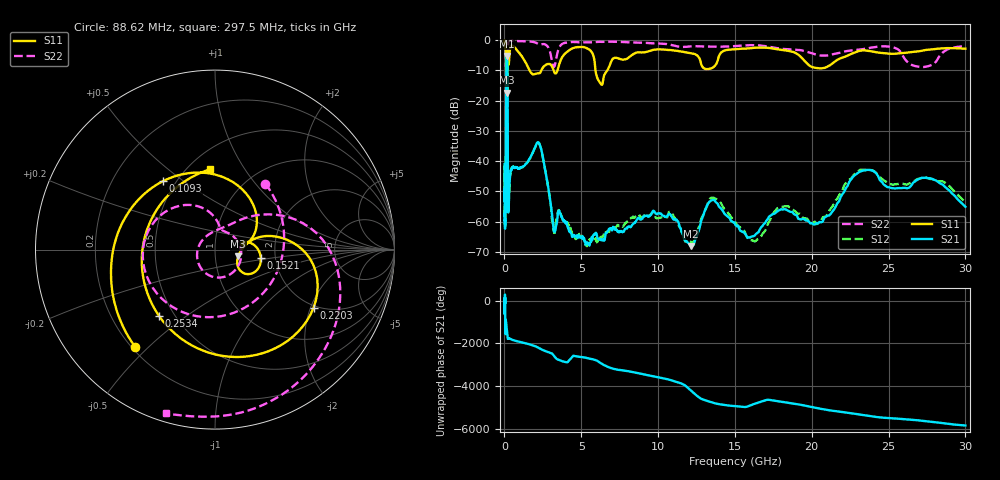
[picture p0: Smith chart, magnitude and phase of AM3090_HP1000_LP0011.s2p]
! Date/Time: Thu, Feb 28, 2019 2:01 PM
! Network Analyzer: Agilent Technologies E8364B Rev: A.07.50.67
! Sweep from 0.010 to 30.000 GHz, 1601 Points, Sweep Type: LOG
! Power Supply: 5.023 V, 0.002 A
# Hz S DB R 50
!freq MagS11 AngS11 MagS21 AngS21 MagS12 AngS12 MagS22 AngS22
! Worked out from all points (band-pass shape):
!   1601 points, 10 MHz to 30 GHz, reference 50 ohm
!   highest |S21| = -5.32 dB at 149.9 MHz (marker M1); lowest = -68.0 dB at 12.13 GHz (marker M2)
!   |S21| within 3 dB of the highest: 121.5 MHz to 190.9 MHz (69.33 MHz wide, 44.4 % of centre)
!   lowest |S11| = -17.4 dB at 185.8 MHz (marker M3), VSWR 1.31, Z = 64.7 - j4.81 ohm
!   |S11| at or under -10 dB: 1.623 GHz to 2.401 GHz (778.5 MHz wide, 38.7 % of centre); 3.196 GHz to 3.454 GHz (258 MHz wide, 7.76 % of centre); 5.925 GHz to 6.698 GHz (772.4 MHz wide, 12.2 % of centre)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
!   |S22| runs from -21.1 to -0.2 dB; largest |S21 - S12| = 0.013
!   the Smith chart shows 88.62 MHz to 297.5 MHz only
!   S11 on the Smith chart (normalised r, x): 88.62 MHz: 0.21, -0.45; 109.3 MHz: 0.43, +0.42; 152.1 MHz: 1.68, -0.17; 220.3 MHz: 1.93, -2.10; 253.4 MHz: 0.41, -0.40; 297.5 MHz: 0.63, +0.71
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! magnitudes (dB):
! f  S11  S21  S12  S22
! 10 MHz  -0.3  -41.0  -43.1  -0.6
! 38.04 MHz  -0.5  -60.2  -58.7  -1.4
! 88.62 MHz  -3.1  -48.6  -49.8  -6.7
! 109.3 MHz  -6.4  -19.1  -19.1  -7.8
! 144.7 MHz  -12.8  -5.4  -5.3  -17.3
! 149.9 MHz  -11.9  -5.3  -5.3  -16.4
! 152.1 MHz  -11.7  -5.3  -5.3  -16.1
! 185.8 MHz  -17.4  -7.2  -7.2  -20.3
! 201.3 MHz  -10.8  -14.3  -14.3  -11.5
! 220.3 MHz  -3.9  -43.6  -43.3  -2.8
! 253.4 MHz  -6.3  -56.0  -54.5  -0.8
! 297.5 MHz  -7.0  -51.5  -51.9  -0.4
! 550.5 MHz  -2.0  -41.9  -42.1  -0.3
! 2.084 GHz  -11.1  -34.3  -34.4  -1.0
! 3.204 GHz  -10.1  -62.9  -62.6  -8.9
! 7.926 GHz  -6.3  -62.3  -60.3  -0.7
! 12.13 GHz  -4.4  -68.0  -66.6  -2.1
! 13.61 GHz  -8.9  -52.9  -52.1  -2.2
! 16.21 GHz  -2.6  -64.8  -66.3  -1.7
! 20.41 GHz  -9.3  -60.6  -60.5  -5.0
! 23.36 GHz  -3.4  -43.1  -42.8  -3.0
! 30 GHz  -2.9  -55.1  -53.5  -2.2
